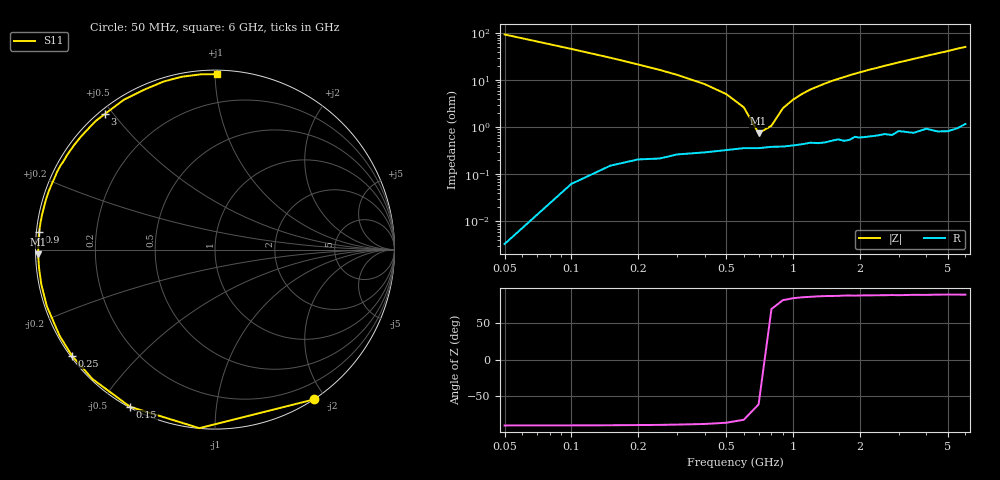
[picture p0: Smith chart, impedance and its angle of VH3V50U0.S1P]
! Infineon Technologies  Discrete & RF Semiconductors
! BB 814
! Si Tuning Diode in SOT23
! VR = 3.5 V
! S-Parameters:  July  1999
# GHz  S  MA  R  50
!  f  S11
! GHz  MAG  ANG
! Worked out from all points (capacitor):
!   34 points, 50 MHz to 6 GHz, reference 50 ohm
!   read as one part to ground: C = 34.1 pF near 50 MHz
!   lowest |Z| = 747 mohm at 700 MHz (marker M1)
!   series resonance near 739.5 MHz, so ESL is about 1.4 nH
!   S11 on the Smith chart (normalised r, x): 50 MHz: 0.00, -1.86; 150 MHz: 0.00, -0.60; 250 MHz: 0.00, -0.33; 900 MHz: 0.01, +0.05; 3 GHz: 0.02, +0.47; 6 GHz: 0.02, +1.01
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0.05  1 -56.6
0.1  0.9986 -95.0
0.15  0.9955 -118.4
0.2  0.993 -133.5
0.25  0.9922 -143.5
0.3  0.9901 -151.0
0.4  0.9887 -161.4
0.5  0.9871 -168.5
0.6  0.9857 -174.0
0.7  0.9857 -178.5
0.8  0.9848 177.7
0.9  0.9846 174.3
1.2  0.9817 165.6
1.4  0.9816 160.7
1.6  0.979 156.1
1.7  0.9806 153.9
1.9  0.977 149.5
2.2  0.9774 143.5
2.4  0.9767 140.0
2.6  0.9757 136.1
2.8  0.9773 132.8
3  0.9733 129.2
3.5  0.9772 121.3
4  0.9743 113.8
4.5  0.9792 107.0
5  0.9806 100.9
5.5  0.9798 94.5
6  0.9771 89.3
